|   stm32f427_437_429_439_ufbga176 IBIS Model
[IBIS ver]   4.2
[File name]  stm32f427_437_429_439_ufbga176.ibs
[File Rev]   1.3
[Date]   05-30-2014
[Source] Data Created at STMicroelectronics
[Notes]   File originated from ELDO simulations.
[Disclaimer]  This information is for modeling purpose only and is
   not guaranted. The information is subject to change without
   notice.
[Copyright] Copyright 2014 STMicroelectronics Inc.
[Component] stm32f427_437_429_439_ufbga176
[Manufacturer] STMicroelectronics
[Package]
| variable   typ   min   max
R_pkg   0.0   NA   NA
L_pkg   0.0H   NA   NA
C_pkg   0.0F   NA   NA
[Pin]   signal_name   model_name   R_pin   L_pin   C_pin
A2 PE2 io8p_arsudq_ft
A1 PE3 io8p_arsudq_ft
B1 PE4 io8p_arsudq_ft
B2 PE5 io8p_arsudq_ft
B3 PE6 io8p_arsudq_ft
C1 VBAT POWER
D2 PI8 io8p_arsudq_ft_v33
D1 PC13 io8p_arwsudq_ft_v33
E1 PC14 io8p_arwsudq_ft
F1 PC15 io8p_arsudq_ft
D3 PI9 io8p_arsudq_ft
E3 PI10 io8p_arsudq_ft
E4 PI11 io8p_arsudq_ft
F2 VSS GND
F3 VDD POWER
E2 PF0 io8p_arsudq_i2cin_ft
H3 PF1 io8p_arsudq_i2cin_ft
H2 PF2 io8p_arsudq_ft
J2 PF3 io8p_arwsudq_ft
J3 PF4 io8p_arwsudq_ft
K3 PF5 io8p_arwsudq_ft
G2 VSS GND
G3 VDD POWER
K2 PF6 io8p_arwsudq_ft
K1 PF7 io8p_arwsudq_ft
L3 PF8 io8p_arwsudq_ft
L2 PF9 io8p_arwsudq_ft
L1 PF10 io8p_arwsudq_ft
G1 PH0 io8p_arsudq_ft
H1 PH1 io8p_arsudq_ft
J1 NRST ioreset_ft_v33
M2 PC0 io8p_ar3wsudq_ft
M3 PC1 io8p_ar3wsudq_ft
M4 PC2 io8p_ar3wsudq_ft
M5 PC3 io8p_ar3wsudq_ft
M1 VSSA GND
N1 VREF- GND
P1 VREF+ POWER
R1 VDDA POWER
N3 PA0 io8p_ar3wsudq_ft_v33
N2 PA1 io8p_ar3wsudq_ft
P2 PA2 io8p_ar3wsudq_ft
F4 PH2 io8p_arsudq_ft
G4 PH3 io8p_arsudq_ft
H4 PH4 io8p_arsudq_i2cin_ft
J4 PH5 io8p_arsudq_i2cin_ft
R2 PA3 io8p_ar3wsudq_ft
L4 BYPASS_REG io8p_arsudq_ft_v33
K4 VDD POWER
N4 PA4 io8p_ar3wsudq_ft
P4 PA5 io8p_ar3wsudq_ft
P3 PA6 io8p_ar3wsudq_ft
R3 PA7 io8p_ar3wsudq_ft
N5 PC4 io8p_ar3wsudq_ft
P5 PC5 io8p_ar3wsudq_ft
R5 PB0 io8p_ar3wsudq_ft
R4 PB1 io8p_ar3wsudq_ft
M6 PB2 io8p_ar3wsudq_ft
R6 PF11 io8p_arsudq_ft
P6 PF12 io8p_arsudq_ft
M8 VSS GND
N8 VDD POWER
N6 PF13 io8p_arsudq_ft
R7 PF14 io8p_arsudq_ft
P7 PF15 io8p_arsudq_ft
N7 PG0 io8p_arsudq_ft
M7 PG1 io8p_arsudq_ft
R8 PE7 io8p_arsudq_ft
P8 PE8 io8p_arsudq_ft
P9 PE9 io8p_arsudq_ft
M9 VSS GND
N9 VDD POWER
R9 PE10 io8p_arsudq_ft
P10 PE11 io8p_arsudq_ft
R10 PE12 io8p_arsudq_ft
N11 PE13 io8p_arsudq_ft
P11 PE14 io8p_arsudq_ft
R11   PE15   io8p_ar3wsudq_ft
R12   PB10   io8p_arsudq_i2cin_ft
R13   PB11   io8p_arsudq_i2cin_ft
L11   VCAP1   POWER
N10 VDD POWER
M11 PH6 io8p_arsudq_ft
N12 PH7 io8p_arsudq_i2cin_ft
M12 PH8 io8p_arsudq_i2cin_ft
M13 PH9 io8p_arsudq_ft
L13 PH10 io8p_arsudq_ft
L12 PH11 io8p_arsudq_ft
K12 PH12 io8p_arsudq_ft
H12 VSS GND
J12 VDD POWER
P12 PB12 io8usb_id_otg_ft
P13 PB13 io8usb_vbus_otg_ft
R14 PB14 io8usb_lsfs_otg_ft
R15 PB15 io8usb_lsfs_otg_ft
P15 PD8 io8p_arsudq_ft
P14 PD9 io8p_arsudq_ft
N15 PD10 io8p_arsudq_ft
N14 PD11 io8p_arsudq_ft
N13 PD12 io8p_arsudq_ft
M15 PD13 io8p_arsudq_ft
J13 VDD POWER
M14 PD14 io8p_arsudq_ft
L14 PD15 io8p_arsudq_ft
L15 PG2 io8p_arsudq_ft
K15 PG3 io8p_arsudq_ft
K14 PG4 io8p_arsudq_ft
K13 PG5 io8p_arsudq_ft
J15 PG6 io8p_arsudq_ft
J14 PG7 io8p_arsudq_ft
H14 PG8 io8p_arsudq_ft
G12 VSS GND
H13 VDD POWER
H15 PC6 io8p_arsudq_ft
G15 PC7 io8p_arsudq_ft
G14 PC8 io8p_arsudq_ft
F14 PC9 io8p_arsudq_i2cin_ft
F15 PA8 io8p_arsudq_i2cin_ft
E15 PA9 io8usb_vbus_otg_ft
D15 PA10 io8usb_id_otg_ft
C15 PA11 io8usb_lsfs_otg_ft
B15 PA12 io8usb_lsfs_otg_ft
A15 PA13 io8p_arsudq_ft
F13 VCAP2 POWER
F12 VSS GND
G13 VDD POWER
E12 PH13 io8p_arsudq_ft
E13 PH14 io8p_arsudq_ft
D13 PH15 io8p_arsudq_ft
E14 PI0 io8p_arsudq_ft
D14 PI1 io8p_arsudq_ft
C14 PI2 io8p_arsudq_ft
C13 PI3 io8p_arsudq_ft
D9 VSS GND
C9 VDD POWER
A14 PA14 io8p_arsudq_ft
A13   PA15   io8p_arsudq_ft
B14 PC10 io8p_arsudq_ft
B13 PC11 io8p_arsudq_ft
A12 PC12 io8p_arsudq_ft
B12 PD0 io8p_arsudq_ft
C12 PD1 io8p_arsudq_ft
D12 PD2 io8p_arsudq_ft
D11 PD3 io8p_arsudq_ft
D10 PD4 io8p_arsudq_ft
C11 PD5 io8p_arsudq_ft
D8 VSS GND
C8 VDD POWER
B11 PD6 io8p_arsudq_ft
A11 PD7 io8p_arsudq_ft
C10 PG9 io8p_arsudq_ft
B10 PG10 io8p_arsudq_ft
B9 PG11 io8p_arsudq_ft
B8 PG12 io8p_arsudq_ft
A8 PG13 io8p_arsudq_ft
A7 PG14 io8p_arsudq_ft
D7 VSS GND
C7 VDD POWER
B7 PG15 io8p_arsudq_ft
A10 PB3 io8p_arsudq_ft
A9 PB4 io8p_arsudq_ft
A6 PB5 io8p_ar3wsudq_ft
B6 PB6 io8p_arsudq_i2cin_ft
B5 PB7 io8p_arsudq_i2cin_ft
D6 BOOT0 vpp_test_hv
A5 PB8 io8p_arsudq_i2cin_ft
B4 PB9 io8p_arsudq_i2cin_ft
A4 PE0 io8p_arsudq_ft
A3 PE1 io8p_arsudq_ft
D5 VSS GND
C6 PDR_ON io8p_arsudq_ft_v33
C5 VDD POWER
D4 PI4 io8p_arsudq_ft
C4 PI5 io8p_arsudq_ft
C3 PI6 io8p_arsudq_ft
C2 PI7 io8p_arsudq_ft
[Diff Pin]   inv_pin   vdiff   tdelay_typ  tdelay_min  tdelay_max
R14   R15   200mV   NA   NA   NA
B15   C15   200mV   NA   NA   NA
[Model Selector] io8p_ar3wsudq_ft
io8p00_ar3wsudq_ft_pd_lv  "SPEED00 1P8V, PD=40kOhm"
io8p00_ar3wsudq_ft_pu_lv  "SPEED00 1P8V, PU=40kOhm"
io8p00_ar3wsudq_ft_lv   "SPEED00 1P8V"
io8p01_ar3wsudq_ft_pd_lv  "SPEED01 1P8V, PD=40kOhm"
io8p01_ar3wsudq_ft_pu_lv  "SPEED01 1P8V, PU=40kOhm"
io8p01_ar3wsudq_ft_lv  "SPEED01 1P8V"
io8p10_ar3wsudq_ft_pd_lv  "SPEED10 1P8V, PD=40kOhm"
io8p10_ar3wsudq_ft_pu_lv  "SPEED10 1P8V, PU=40kOhm"
io8p10_ar3wsudq_ft_lv  "SPEED10 1P8V"
io8p11_ar3wsudq_ft_pd_lv  "SPEED11 1P8V, PD=40kOhm"
io8p11_ar3wsudq_ft_pu_lv  "SPEED11 1P8V, PU=40kOhm"
io8p11_ar3wsudq_ft_lv  "SPEED11 1P8V"
io8p00_ar3wsudq_ft_pd  "SPEED00, PD=40kOhm"
io8p00_ar3wsudq_ft_pu  "SPEED00, PU=40kOhm"
io8p00_ar3wsudq_ft  "SPEED00"
io8p01_ar3wsudq_ft_pd  "SPEED01, PD=40kOhm"
io8p01_ar3wsudq_ft_pu  "SPEED01, PU=40kOhm"
io8p01_ar3wsudq_ft  "SPEED01"
io8p10_ar3wsudq_ft_pd  "SPEED10, PD=40kOhm"
io8p10_ar3wsudq_ft_pu  "SPEED10, PU=40kOhm"
io8p10_ar3wsudq_ft  "SPEED10"
io8p11_ar3wsudq_ft_pd  "SPEED11, PD=40kOhm"
io8p11_ar3wsudq_ft_pu  "SPEED11, PU=40kOhm"
io8p11_ar3wsudq_ft  "SPEED11"
[Model Selector] io8p_ar3wsudq_ft_v33
io8p00_ar3wsudq_ft_v33_pd_lv  "SPEED00 1P8V, PD=40kOhm"
io8p00_ar3wsudq_ft_v33_pu_lv  "SPEED00 1P8V, PU=40kOhm"
io8p00_ar3wsudq_ft_v33_lv  "SPEED00 1P8V"
io8p01_ar3wsudq_ft_v33_pd_lv  "SPEED01 1P8V, PD=40kOhm"
io8p01_ar3wsudq_ft_v33_pu_lv  "SPEED01 1P8V, PU=40kOhm"
io8p01_ar3wsudq_ft_v33_lv  "SPEED01 1P8V"
io8p10_ar3wsudq_ft_v33_pd_lv  "SPEED10 1P8V, PD=40kOhm"
io8p10_ar3wsudq_ft_v33_pu_lv  "SPEED10 1P8V, PU=40kOhm"
io8p10_ar3wsudq_ft_v33_lv  "SPEED10 1P8V"
io8p11_ar3wsudq_ft_v33_pd_lv  "SPEED11 1P8V, PD=40kOhm"
io8p11_ar3wsudq_ft_v33_pu_lv  "SPEED11 1P8V, PU=40kOhm"
io8p11_ar3wsudq_ft_v33_lv  "SPEED11 1P8V"
io8p00_ar3wsudq_ft_v33_pd  "SPEED00, PD=40kOhm"
io8p00_ar3wsudq_ft_v33_pu  "SPEED00, PU=40kOhm"
io8p00_ar3wsudq_ft_v33  "SPEED00"
io8p01_ar3wsudq_ft_v33_pd  "SPEED01, PD=40kOhm"
io8p01_ar3wsudq_ft_v33_pu  "SPEED01, PU=40kOhm"
io8p01_ar3wsudq_ft_v33  "SPEED01"
io8p10_ar3wsudq_ft_v33_pd  "SPEED10, PD=40kOhm"
io8p10_ar3wsudq_ft_v33_pu  "SPEED10, PU=40kOhm"
io8p10_ar3wsudq_ft_v33  "SPEED10"
io8p11_ar3wsudq_ft_v33_pd  "SPEED11, PD=40kOhm"
io8p11_ar3wsudq_ft_v33_pu  "SPEED11, PU=40kOhm"
io8p11_ar3wsudq_ft_v33  "SPEED11"
[Model Selector] io8p_arsudq_ft
io8p00_arsudq_ft_pd_lv  "SPEED00 1P8V, PD=40kOhm"
io8p00_arsudq_ft_pu_lv  "SPEED00 1P8V, PU=40kOhm"
io8p00_arsudq_ft_lv  "SPEED00 1P8V"
io8p01_arsudq_ft_pd_lv  "SPEED01 1P8V, PD=40kOhm"
io8p01_arsudq_ft_pu_lv  "SPEED01 1P8V, PU=40kOhm"
io8p01_arsudq_ft_lv  "SPEED01 1P8V"
io8p10_arsudq_ft_pd_lv  "SPEED10 1P8V, PD=40kOhm"
io8p10_arsudq_ft_pu_lv  "SPEED10 1P8V, PU=40kOhm"
io8p10_arsudq_ft_lv  "SPEED10 1P8V"
io8p11_arsudq_ft_pd_lv  "SPEED11 1P8V, PD=40kOhm"
io8p11_arsudq_ft_pu_lv  "SPEED11 1P8V, PU=40kOhm"
io8p11_arsudq_ft_lv  "SPEED11 1P8V"
io8p00_arsudq_ft_pd  "SPEED00, PD=40kOhm"
io8p00_arsudq_ft_pu  "SPEED00, PU=40kOhm"
io8p00_arsudq_ft  "SPEED00"
io8p01_arsudq_ft_pd  "SPEED01, PD=40kOhm"
io8p01_arsudq_ft_pu  "SPEED01, PU=40kOhm"
io8p01_arsudq_ft  "SPEED01"
io8p10_arsudq_ft_pd  "SPEED10, PD=40kOhm"
io8p10_arsudq_ft_pu  "SPEED10, PU=40kOhm"
io8p10_arsudq_ft  "SPEED10"
io8p11_arsudq_ft_pd  "SPEED11, PD=40kOhm"
io8p11_arsudq_ft_pu  "SPEED11, PU=40kOhm"
io8p11_arsudq_ft  "SPEED11"
[Model Selector] io8p_arsudq_ft_v33
io8p00_arsudq_ft_v33_pd_lv  "SPEED00 1P8V, PD=40kOhm"
io8p00_arsudq_ft_v33_pu_lv  "SPEED00 1P8V, PU=40kOhm"
io8p00_arsudq_ft_v33_lv  "SPEED00 1P8V"
io8p01_arsudq_ft_v33_pd_lv  "SPEED01 1P8V, PD=40kOhm"
io8p01_arsudq_ft_v33_pu_lv  "SPEED01 1P8V, PU=40kOhm"
io8p01_arsudq_ft_v33_lv  "SPEED01 1P8V"
io8p10_arsudq_ft_v33_pd_lv  "SPEED10 1P8V, PD=40kOhm"
io8p10_arsudq_ft_v33_pu_lv  "SPEED10 1P8V, PU=40kOhm"
io8p10_arsudq_ft_v33_lv  "SPEED10 1P8V"
io8p11_arsudq_ft_v33_pd_lv  "SPEED11 1P8V, PD=40kOhm"
io8p11_arsudq_ft_v33_pu_lv  "SPEED11 1P8V, PU=40kOhm"
io8p11_arsudq_ft_v33_lv  "SPEED11 1P8V"
io8p00_arsudq_ft_v33_pd  "SPEED00, PD=40kOhm"
io8p00_arsudq_ft_v33_pu  "SPEED00, PU=40kOhm"
io8p00_arsudq_ft_v33  "SPEED00"
io8p01_arsudq_ft_v33_pd  "SPEED01, PD=40kOhm"
io8p01_arsudq_ft_v33_pu  "SPEED01, PU=40kOhm"
io8p01_arsudq_ft_v33  "SPEED01"
io8p10_arsudq_ft_v33_pd  "SPEED10, PD=40kOhm"
io8p10_arsudq_ft_v33_pu  "SPEED10, PU=40kOhm"
io8p10_arsudq_ft_v33  "SPEED10"
io8p11_arsudq_ft_v33_pd  "SPEED11, PD=40kOhm"
io8p11_arsudq_ft_v33_pu  "SPEED11, PU=40kOhm"
io8p11_arsudq_ft_v33  "SPEED11"
[Model Selector] io8p_arsudq_i2cin_ft
io8p00_arsudq_i2cin_ft_pd_lv  "SPEED00 1P8V, PD=40kOhm"
io8p00_arsudq_i2cin_ft_pu_lv  "SPEED00 1P8V, PU=40kOhm"
io8p00_arsudq_i2cin_ft_lv  "SPEED00 1P8V"
io8p01_arsudq_i2cin_ft_pd_lv  "SPEED01 1P8V, PD=40kOhm"
io8p01_arsudq_i2cin_ft_pu_lv  "SPEED01 1P8V, PU=40kOhm"
io8p01_arsudq_i2cin_ft_lv  "SPEED01 1P8V"
io8p10_arsudq_i2cin_ft_pd_lv  "SPEED10 1P8V, PD=40kOhm"
io8p10_arsudq_i2cin_ft_pu_lv  "SPEED10 1P8V, PU=40kOhm"
io8p10_arsudq_i2cin_ft_lv  "SPEED10 1P8V"
io8p11_arsudq_i2cin_ft_pd_lv  "SPEED11 1P8V, PD=40kOhm"
io8p11_arsudq_i2cin_ft_pu_lv  "SPEED11 1P8V, PU=40kOhm"
io8p11_arsudq_i2cin_ft_lv  "SPEED11 1P8V"
io8p00_arsudq_i2cin_ft_pd  "SPEED00, PD=40kOhm"
io8p00_arsudq_i2cin_ft_pu  "SPEED00, PU=40kOhm"
io8p00_arsudq_i2cin_ft  "SPEED00"
io8p01_arsudq_i2cin_ft_pd  "SPEED01, PD=40kOhm"
io8p01_arsudq_i2cin_ft_pu  "SPEED01, PU=40kOhm"
io8p01_arsudq_i2cin_ft  "SPEED01"
io8p10_arsudq_i2cin_ft_pd  "SPEED10, PD=40kOhm"
io8p10_arsudq_i2cin_ft_pu  "SPEED10, PU=40kOhm"
io8p10_arsudq_i2cin_ft  "SPEED10"
io8p11_arsudq_i2cin_ft_pd  "SPEED11, PD=40kOhm"
io8p11_arsudq_i2cin_ft_pu  "SPEED11, PU=40kOhm"
io8p11_arsudq_i2cin_ft  "SPEED11"
[Model Selector] io8p_arwsudq_ft
io8p00_arwsudq_ft_pd_lv  "SPEED00 1P8V, PD=40kOhm"
io8p00_arwsudq_ft_pu_lv  "SPEED00 1P8V, PU=40kOhm"
io8p00_arwsudq_ft_lv  "SPEED00 1P8V"
io8p01_arwsudq_ft_pd_lv  "SPEED01 1P8V, PD=40kOhm"
io8p01_arwsudq_ft_pu_lv  "SPEED01 1P8V, PU=40kOhm"
io8p01_arwsudq_ft_lv  "SPEED01 1P8V"
io8p10_arwsudq_ft_pd_lv  "SPEED10 1P8V, PD=40kOhm"
io8p10_arwsudq_ft_pu_lv  "SPEED10 1P8V, PU=40kOhm"
io8p10_arwsudq_ft_lv  "SPEED10 1P8V"
io8p11_arwsudq_ft_pd_lv  "SPEED11 1P8V, PD=40kOhm"
io8p11_arwsudq_ft_pu_lv  "SPEED11 1P8V, PU=40kOhm"
io8p11_arwsudq_ft_lv  "SPEED11 1P8V"
io8p00_arwsudq_ft_pd  "SPEED00, PD=40kOhm"
io8p00_arwsudq_ft_pu  "SPEED00, PU=40kOhm"
io8p00_arwsudq_ft  "SPEED00"
io8p01_arwsudq_ft_pd  "SPEED01, PD=40kOhm"
io8p01_arwsudq_ft_pu  "SPEED01, PU=40kOhm"
io8p01_arwsudq_ft  "SPEED01"
io8p10_arwsudq_ft_pd  "SPEED10, PD=40kOhm"
io8p10_arwsudq_ft_pu  "SPEED10, PU=40kOhm"
io8p10_arwsudq_ft  "SPEED10"
io8p11_arwsudq_ft_pd  "SPEED11, PD=40kOhm"
io8p11_arwsudq_ft_pu  "SPEED11, PU=40kOhm"
io8p11_arwsudq_ft  "SPEED11"
[Model Selector] io8p_arwsudq_ft_v33
io8p00_arwsudq_ft_v33_pd_lv  "SPEED00 1P8V, PD=40kOhm"
io8p00_arwsudq_ft_v33_pu_lv  "SPEED00 1P8V, PU=40kOhm"
io8p00_arwsudq_ft_v33_lv  "SPEED00 1P8V"
io8p01_arwsudq_ft_v33_pd_lv  "SPEED01 1P8V, PD=40kOhm"
io8p01_arwsudq_ft_v33_pu_lv  "SPEED01 1P8V, PU=40kOhm"
io8p01_arwsudq_ft_v33_lv  "SPEED01 1P8V"
io8p10_arwsudq_ft_v33_pd_lv  "SPEED10 1P8V, PD=40kOhm"
io8p10_arwsudq_ft_v33_pu_lv  "SPEED10 1P8V, PU=40kOhm"
io8p10_arwsudq_ft_v33_lv  "SPEED10 1P8V"
io8p11_arwsudq_ft_v33_pd_lv  "SPEED11 1P8V, PD=40kOhm"
io8p11_arwsudq_ft_v33_pu_lv  "SPEED11 1P8V, PU=40kOhm"
io8p11_arwsudq_ft_v33_lv  "SPEED11 1P8V"
io8p00_arwsudq_ft_v33_pd  "SPEED00, PD=40kOhm"
io8p00_arwsudq_ft_v33_pu  "SPEED00, PU=40kOhm"
io8p00_arwsudq_ft_v33  "SPEED00"
io8p01_arwsudq_ft_v33_pd  "SPEED01, PD=40kOhm"
io8p01_arwsudq_ft_v33_pu  "SPEED01, PU=40kOhm"
io8p01_arwsudq_ft_v33  "SPEED01"
io8p10_arwsudq_ft_v33_pd  "SPEED10, PD=40kOhm"
io8p10_arwsudq_ft_v33_pu  "SPEED10, PU=40kOhm"
io8p10_arwsudq_ft_v33  "SPEED10"
io8p11_arwsudq_ft_v33_pd  "SPEED11, PD=40kOhm"
io8p11_arwsudq_ft_v33_pu  "SPEED11, PU=40kOhm"
io8p11_arwsudq_ft_v33  "SPEED11"
[Model Selector] io8usb_id_otg_ft
io8p00_id_otg_ft_pd_lv  "SPEED00 1P8V, PD=14kOhm"
io8p00_id_otg_ft_pu_lv  "SPEED00 1P8V, PU=14kOhm"
io8p00_id_otg_ft_lv  "SPEED00 1P8V"
io8p01_id_otg_ft_pd_lv  "SPEED01 1P8V, PD=14kOhm"
io8p01_id_otg_ft_pu_lv  "SPEED01 1P8V, PU=14kOhm"
io8p01_id_otg_ft_lv  "SPEED01 1P8V"
io8p10_id_otg_ft_pd_lv  "SPEED10 1P8V, PD=14kOhm"
io8p10_id_otg_ft_pu_lv  "SPEED10 1P8V, PU=14kOhm"
io8p10_id_otg_ft_lv  "SPEED10 1P8V"
io8p11_id_otg_ft_pd_lv  "SPEED11 1P8V, PD=14kOhm"
io8p11_id_otg_ft_pu_lv  "SPEED11 1P8V, PU=14kOhm"
io8p11_id_otg_ft_lv  "SPEED11 1P8V"
io8p00_id_otg_ft_pd  "SPEED00, PD=14kOhm"
io8p00_id_otg_ft_pu  "SPEED00, PU=14kOhm"
io8p00_id_otg_ft  "SPEED00"
io8p01_id_otg_ft_pd  "SPEED01, PD=14kOhm"
io8p01_id_otg_ft_pu  "SPEED01, PU=14kOhm"
io8p01_id_otg_ft  "SPEED01"
io8p10_id_otg_ft_pd  "SPEED10, PD=14kOhm"
io8p10_id_otg_ft_pu  "SPEED10, PU=14kOhm"
io8p10_id_otg_ft  "SPEED10"
io8p11_id_otg_ft_pd  "SPEED11, PD=14kOhm"
io8p11_id_otg_ft_pu  "SPEED11, PU=14kOhm"
io8p11_id_otg_ft  "SPEED11"
[Model Selector] io8usb_lsfs_otg_ft
io8usb_ls_otg_ft_dpdn_pd  "LS USB DP/DN IO + PD=20kOhm"
io8usb_ls_otg_ft_dpdn_pupu2  "LS USB DP/DN IO + PU/PU2=2.2kOhm"
io8usb_ls_otg_ft_dpdn_pu2  "LS USB DP/DN IO + PU2=1.2kOhm"
io8usb_ls_otg_ft_dpdn_pu  "LS USB DP/DN IO + PU=1.2kOhm"
io8usb_ls_otg_ft_dpdn  "LS USB DP/DN IO"
io8usb_fs_otg_ft_dpdn_pd  "HS USB DP/DN IO + PD=20kOhm"
io8usb_fs_otg_ft_dpdn_pupu2  "HS USB DP/DN IO + PU/PU2=2.2kOhm"
io8usb_fs_otg_ft_dpdn_pu2  "HS USB DP/DN IO + PU2=1.2kOhm"
io8usb_fs_otg_ft_dpdn_pu  "HS USB DP/DN IO + PU=1.2kOhm"
io8usb_fs_otg_ft_dpdn  "HS USB DP/DN IO"
io8p00_lsfs_otg_ft_pd_lv  "SPEED00 1P8V, PD=40kOhm"
io8p00_lsfs_otg_ft_pu_lv  "SPEED00 1P8V, PU=40kOhm"
io8p00_lsfs_otg_ft_lv  "SPEED00 1P8V"
io8p01_lsfs_otg_ft_pd_lv  "SPEED01 1P8V, PD=40kOhm"
io8p01_lsfs_otg_ft_pu_lv  "SPEED01 1P8V, PU=40kOhm"
io8p01_lsfs_otg_ft_lv  "SPEED01 1P8V"
io8p10_lsfs_otg_ft_pd_lv  "SPEED10 1P8V, PD=40kOhm"
io8p10_lsfs_otg_ft_pu_lv  "SPEED10 1P8V, PU=40kOhm"
io8p10_lsfs_otg_ft_lv  "SPEED10 1P8V"
io8p11_lsfs_otg_ft_pd_lv  "SPEED11 1P8V, PD=40kOhm"
io8p11_lsfs_otg_ft_pu_lv  "SPEED11 1P8V, PU=40kOhm"
io8p11_lsfs_otg_ft_lv  "SPEED11 1P8V"
io8p00_lsfs_otg_ft_pd  "SPEED00, PD=40kOhm"
io8p00_lsfs_otg_ft_pu  "SPEED00, PU=40kOhm"
io8p00_lsfs_otg_ft  "SPEED00"
io8p01_lsfs_otg_ft_pd  "SPEED01, PD=40kOhm"
io8p01_lsfs_otg_ft_pu  "SPEED01, PU=40kOhm"
io8p01_lsfs_otg_ft  "SPEED01"
io8p10_lsfs_otg_ft_pd  "SPEED10, PD=40kOhm"
io8p10_lsfs_otg_ft_pu  "SPEED10, PU=40kOhm"
io8p10_lsfs_otg_ft  "SPEED10"
io8p11_lsfs_otg_ft_pd  "SPEED11, PD=40kOhm"
io8p11_lsfs_otg_ft_pu  "SPEED11, PU=40kOhm"
io8p11_lsfs_otg_ft  "SPEED11"
[Model Selector] io8usb_vbus_otg_ft
io8psenb_vbus_otg_ft  "VBUS PULSE, SENSE VB"
io8psenab_vbus_otg_ft  "VBUS PULSE, SENSE VA and VB"
io8psena_vbus_otg_ft  "VBUS PULSE, SENSE VA"
io8psen_vbus_otg_ft  "VBUS PULSE"
io8p00_vbus_otg_ft_pd_lv  "SPEED00 1P8V, PD=40kOhm"
io8p00_vbus_otg_ft_pu_lv  "SPEED00 1P8V, PU=40kOhm"
io8p00_vbus_otg_ft_lv  "SPEED00 1P8V"
io8p01_vbus_otg_ft_pd_lv  "SPEED01 1P8V, PD=40kOhm"
io8p01_vbus_otg_ft_pu_lv  "SPEED01 1P8V, PU=40kOhm"
io8p01_vbus_otg_ft_lv  "SPEED01 1P8V"
io8p10_vbus_otg_ft_pd_lv  "SPEED10 1P8V, PD=40kOhm"
io8p10_vbus_otg_ft_pu_lv  "SPEED10 1P8V, PU=40kOhm"
io8p10_vbus_otg_ft_lv  "SPEED10 1P8V"
io8p11_vbus_otg_ft_pd_lv  "SPEED11 1P8V, PD=40kOhm"
io8p11_vbus_otg_ft_pu_lv  "SPEED11 1P8V, PU=40kOhm"
io8p11_vbus_otg_ft_lv  "SPEED11 1P8V"
io8p00_vbus_otg_ft_pd  "SPEED00, PD=40kOhm"
io8p00_vbus_otg_ft_pu  "SPEED00, PU=40kOhm"
io8p00_vbus_otg_ft  "SPEED00"
io8p01_vbus_otg_ft_pd  "SPEED01, PD=40kOhm"
io8p01_vbus_otg_ft_pu  "SPEED01, PU=40kOhm"
io8p01_vbus_otg_ft  "SPEED01"
io8p10_vbus_otg_ft_pd  "SPEED10, PD=40kOhm"
io8p10_vbus_otg_ft_pu  "SPEED10, PU=40kOhm"
io8p10_vbus_otg_ft  "SPEED10"
io8p11_vbus_otg_ft_pd  "SPEED11, PD=40kOhm"
io8p11_vbus_otg_ft_pu  "SPEED11, PU=40kOhm"
io8p11_vbus_otg_ft  "SPEED11"
[Model Selector] ioreset_ft_v33
ioreset_ft_v33_pu_lv  "ioreset 1P8V + PU=40kOhm"
ioreset_ft_v33_nopu_lv  "ioreset 1P8V"
ioreset_ft_v33_pu  "ioreset + PU=40kOhm"
ioreset_ft_v33_nopu  "ioreset"
[Model Selector] vpp_test_hv
vpp_test_hv_2p4  "Input Buffer 1P8V"
vpp_test_hv_3p3  "Input Buffer"
| Models and submodels in the file (260): io8p00_ar3wsudq_ft_pd_lv (I/O), io8p00_ar3wsudq_ft_pu_lv (I/O), io8p00_ar3wsudq_ft_lv (I/O), io8p01_ar3wsudq_ft_pd_lv (I/O), io8p01_ar3wsudq_ft_pu_lv (I/O), io8p01_ar3wsudq_ft_lv (I/O), io8p10_ar3wsudq_ft_pd_lv (I/O), io8p10_ar3wsudq_ft_pu_lv (I/O), io8p10_ar3wsudq_ft_lv (I/O), io8p11_ar3wsudq_ft_pd_lv (I/O), io8p11_ar3wsudq_ft_pu_lv (I/O), io8p11_ar3wsudq_ft_lv (I/O), io8p00_ar3wsudq_ft_pd (I/O), io8p00_ar3wsudq_ft_pu (I/O), io8p00_ar3wsudq_ft (I/O), io8p01_ar3wsudq_ft_pd (I/O), io8p01_ar3wsudq_ft_pu (I/O), io8p01_ar3wsudq_ft (I/O), io8p10_ar3wsudq_ft_pd (I/O), io8p10_ar3wsudq_ft_pu (I/O), io8p10_ar3wsudq_ft (I/O), io8p11_ar3wsudq_ft_pd (I/O), io8p11_ar3wsudq_ft_pu (I/O), io8p11_ar3wsudq_ft (I/O), io8p00_ar3wsudq_ft_v33_pd_lv (I/O), io8p00_ar3wsudq_ft_v33_pu_lv (I/O), io8p00_ar3wsudq_ft_v33_lv (I/O), io8p01_ar3wsudq_ft_v33_pd_lv (I/O), io8p01_ar3wsudq_ft_v33_pu_lv (I/O), io8p01_ar3wsudq_ft_v33_lv (I/O), io8p10_ar3wsudq_ft_v33_pd_lv (I/O), io8p10_ar3wsudq_ft_v33_pu_lv (I/O), io8p10_ar3wsudq_ft_v33_lv (I/O), io8p11_ar3wsudq_ft_v33_pd_lv (I/O), io8p11_ar3wsudq_ft_v33_pu_lv (I/O), io8p11_ar3wsudq_ft_v33_lv (I/O), io8p00_ar3wsudq_ft_v33_pd (I/O), io8p00_ar3wsudq_ft_v33_pu (I/O), io8p00_ar3wsudq_ft_v33 (I/O), io8p01_ar3wsudq_ft_v33_pd (I/O), io8p01_ar3wsudq_ft_v33_pu (I/O), io8p01_ar3wsudq_ft_v33 (I/O), io8p10_ar3wsudq_ft_v33_pd (I/O), io8p10_ar3wsudq_ft_v33_pu (I/O), io8p10_ar3wsudq_ft_v33 (I/O), io8p11_ar3wsudq_ft_v33_pd (I/O), io8p11_ar3wsudq_ft_v33_pu (I/O), io8p11_ar3wsudq_ft_v33 (I/O), io8p00_arsudq_ft_pd_lv (I/O), io8p00_arsudq_ft_pu_lv (I/O), io8p00_arsudq_ft_lv (I/O), io8p01_arsudq_ft_pd_lv (I/O), io8p01_arsudq_ft_pu_lv (I/O), io8p01_arsudq_ft_lv (I/O), io8p10_arsudq_ft_pd_lv (I/O), io8p10_arsudq_ft_pu_lv (I/O), io8p10_arsudq_ft_lv (I/O), io8p11_arsudq_ft_pd_lv (I/O), io8p11_arsudq_ft_pu_lv (I/O), io8p11_arsudq_ft_lv (I/O), io8p00_arsudq_ft_pd (I/O), io8p00_arsudq_ft_pu (I/O), io8p00_arsudq_ft (I/O), io8p01_arsudq_ft_pd (I/O), io8p01_arsudq_ft_pu (I/O), io8p01_arsudq_ft (I/O), io8p10_arsudq_ft_pd (I/O), io8p10_arsudq_ft_pu (I/O), io8p10_arsudq_ft (I/O), io8p11_arsudq_ft_pd (I/O), io8p11_arsudq_ft_pu (I/O), io8p11_arsudq_ft (I/O), io8p00_arsudq_ft_v33_pd_lv (I/O), io8p00_arsudq_ft_v33_pu_lv (I/O), io8p00_arsudq_ft_v33_lv (I/O), io8p01_arsudq_ft_v33_pd_lv (I/O), io8p01_arsudq_ft_v33_pu_lv (I/O), io8p01_arsudq_ft_v33_lv (I/O), io8p10_arsudq_ft_v33_pd_lv (I/O), io8p10_arsudq_ft_v33_pu_lv (I/O)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
